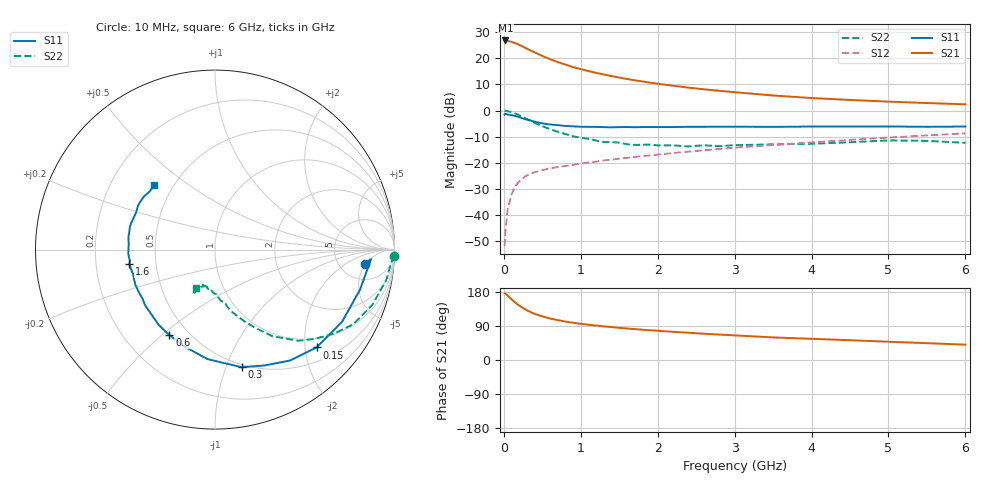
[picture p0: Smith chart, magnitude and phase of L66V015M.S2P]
!  INFINEON TECHNOLOGIES Small Signal Semiconductors
! BFR380L3 , Si-NPN RF-Transistor in TSLP-3-1
!  Vce=6 V,  Ic=15 mA
! Common Emitter S-Parameters:  07. March 2005
#  GHz  S  MA  R  50
! f  S11  S21  S12  S22
! GHz  Mag  Ang  Mag  Ang  Mag  Ang  Mag  Ang
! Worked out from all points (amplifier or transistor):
!   36 points, 10 MHz to 6 GHz, reference 50 ohm
!   highest |S21| = 26.9 dB at 20 MHz (marker M1)
!   |S21| within 3 dB of that: start of sweep to 290.1 MHz
!   unconditionally stable (mu >= 1): 2.594 GHz to 4.663 GHz
!   at 250 MHz: K = 0.26, MSG = 25.2 dB, |S12| = -25.9 dB
!   at 1.4 GHz: K = 0.86, MSG = 16.0 dB, |S12| = -18.9 dB
!   at 6 GHz: K = 0.96, MSG = 5.6 dB, |S12| = -8.7 dB
!   S11 on the Smith chart (normalised r, x): 10 MHz: 8.81, -4.63; 150 MHz: 0.79, -2.25; 300 MHz: 0.48, -1.14; 600 MHz: 0.39, -0.53; 1.6 GHz: 0.35, -0.07; 6 GHz: 0.39, +0.37
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0.01  0.837 -5.4  22.04 175.9  0.0025 69.7  0.9992 -2.0
0.02  0.871 -3.5  22.08 175.8  0.0046 82.0  0.985 -4.1
0.05  0.8385 -15.3  21.66 169.7  0.0127 82.0  0.9696 -10.0
0.1  0.8143 -29.6  20.75 160.3  0.0246 74.5  0.9293 -19.4
0.15  0.7858 -43.9  19.61 151.3  0.0358 68.1  0.8754 -28.4
0.2  0.7458 -56.0  18.18 143.5  0.0435 64.6  0.8127 -35.1
0.25  0.7027 -66.7  16.76 137.1  0.0507 59.6  0.7439 -42.0
0.3  0.672 -77.2  15.36 131.0  0.0569 56.9  0.6888 -47.5
0.4  0.6118 -93.8  13.04 121.8  0.0654 52.4  0.5798 -56.4
0.5  0.5674 -107.0  11.17 115.1  0.0719 50.5  0.5002 -61.9
0.6  0.5398 -118.1  9.655 109.4  0.0776 49.3  0.4406 -67.0
0.7  0.5242 -126.7  8.516 105.2  0.0823 49.4  0.3914 -71.3
0.8  0.5055 -134.6  7.6 101.4  0.0865 49.3  0.3536 -75.5
1.1  0.4864 -151.3  5.711 93.0  0.1006 51.4  0.287 -83.3
1.4  0.476 -163.3  4.568 86.9  0.114 53.2  0.2477 -89.0
1.6  0.4833 -170.4  4.032 83.1  0.1238 54.4  0.2258 -95.7
2.2  0.482 176.1  2.988 74.4  0.1529 57.3  0.2149 -101.4
2.8  0.4905 165.0  2.39 67.1  0.1827 59.2  0.2068 -109.3
3.5  0.4856 155.0  1.94 59.6  0.2177 59.2  0.2242 -111.8
4.5  0.4944 147.5  1.594 52.2  0.2734 59.8  0.2462 -114.3
5.5  0.4874 138.6  1.391 44.4  0.3333 57.8  0.2618 -115.8
6  0.4929 133.2  1.316 40.5  0.3653 56.4  0.2396 -116.5
